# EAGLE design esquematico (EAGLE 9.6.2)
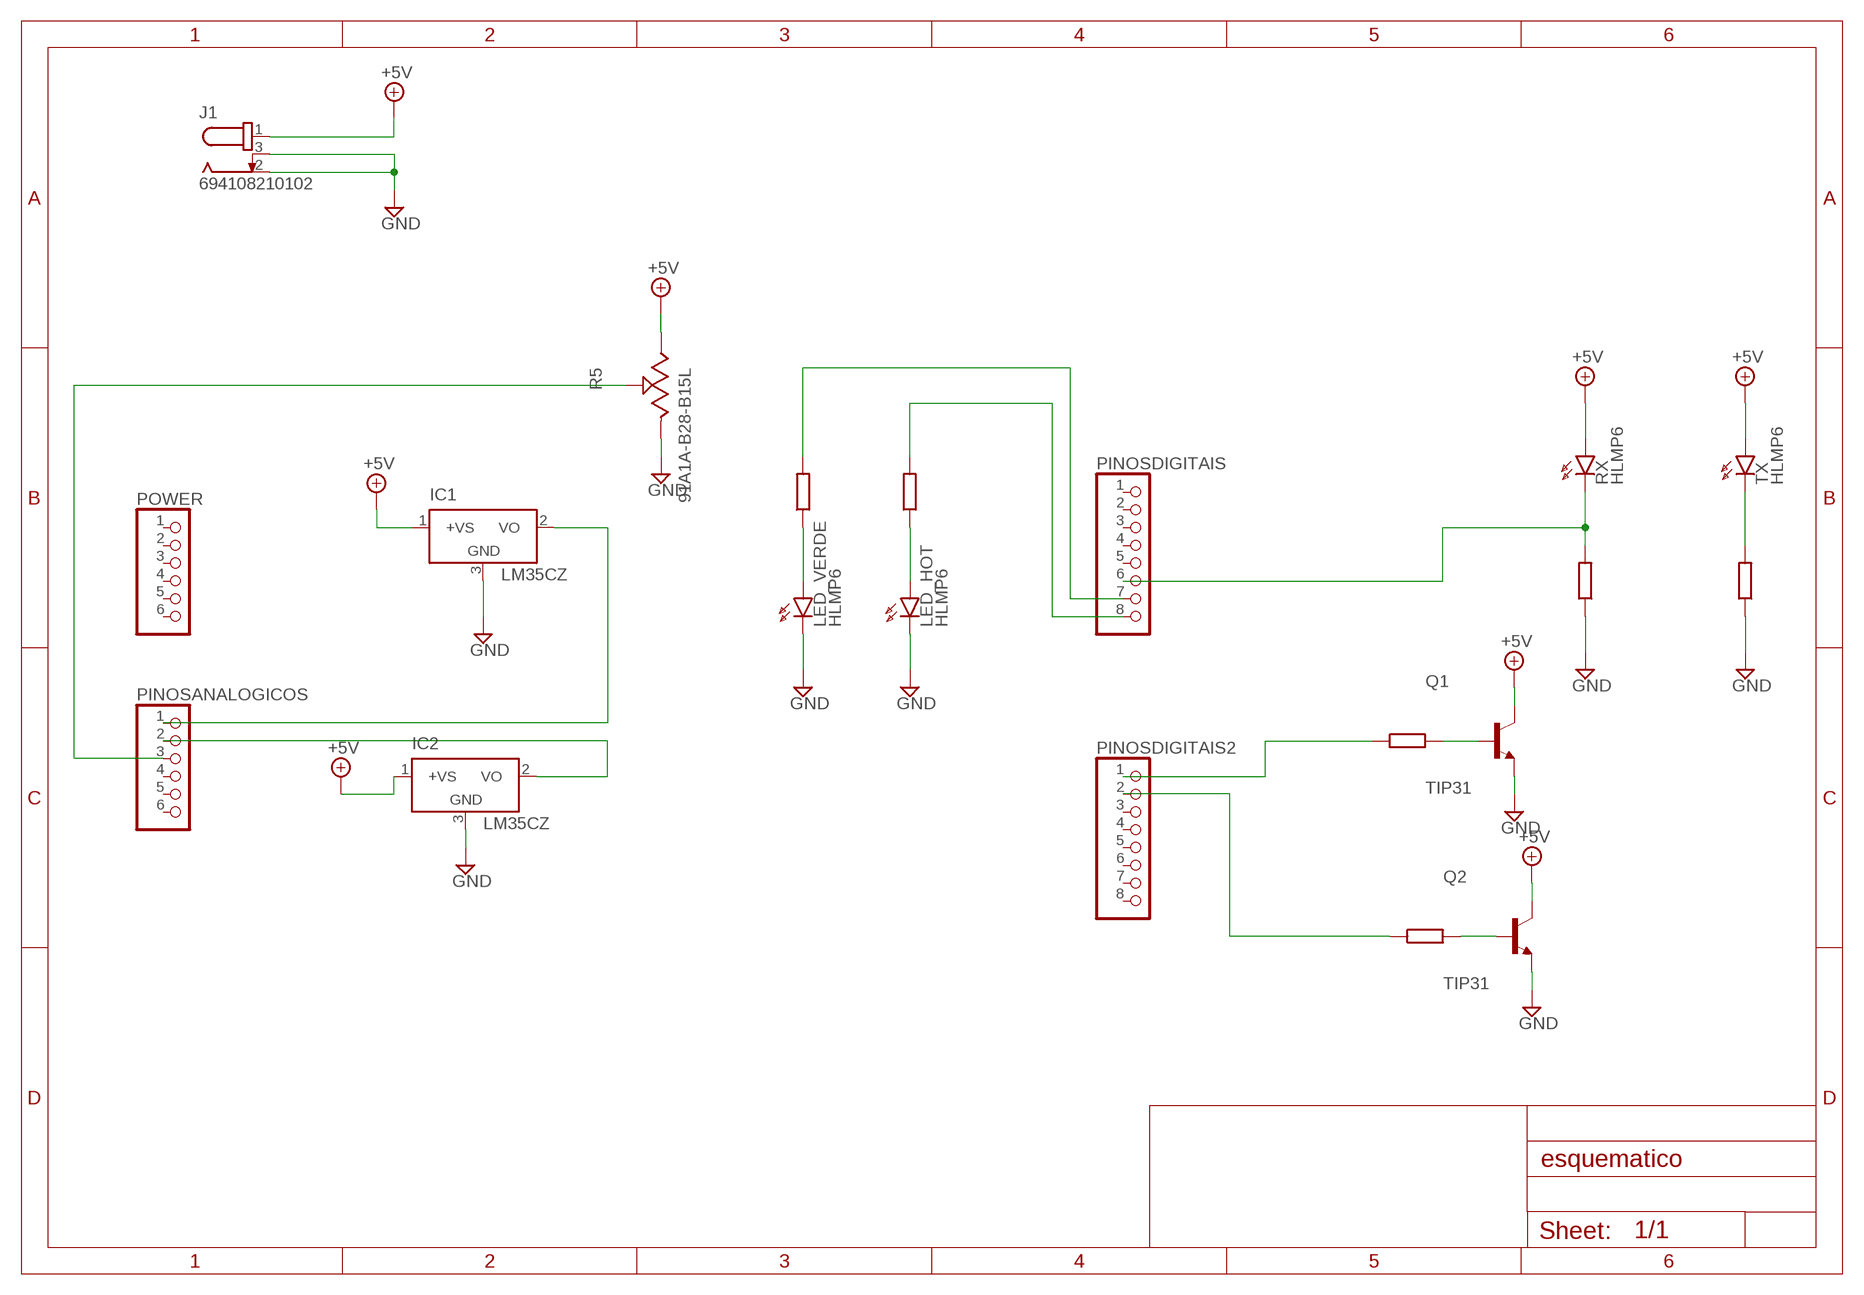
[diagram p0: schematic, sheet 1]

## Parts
IC1  LM35CZ  [TO92]
IC2  LM35CZ  [TO92]
J1  694108210102  [694108210102]
LED_HOT  HLMP6  [HLMP6]
LED_VERDE  HLMP6  [HLMP6]
PINOSANALOGICOS  PINHD-1X6  [1X06]
PINOSDIGITAIS  PINHD-1X8  [1X08]
PINOSDIGITAIS2  PINHD-1X8  [1X08]
POWER  PINHD-1X6  [1X06]
Q1  TIP31  [TO254P1060X482X2222-3]
Q2  TIP31  [TO254P1060X482X2222-3]
R5  91A1A-B28-B15L  [91A1A-B28-B15L-ND]
RX  HLMP6  [HLMP6]
TX  HLMP6  [HLMP6]

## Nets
+5V: IC1.1(+VS) IC2.1(+VS) J1.1 Q1.2(C) Q2.2(C) R5.3 RX.A TX.A
GND: IC1.3(GND) IC2.3(GND) J1.2 J1.3 LED_HOT.K LED_VERDE.K Q1.3(E) Q2.3(E) R5.1
N$1: IC2.2(VO) PINOSANALOGICOS.2
N$2: Q1.1(B)
N$3: LED_HOT.A
N$4: LED_VERDE.A
N$5: IC1.2(VO) PINOSANALOGICOS.1
N$6: Q2.1(B)
N$7: PINOSDIGITAIS2.1
N$8: PINOSDIGITAIS2.2
N$9: PINOSDIGITAIS.6 RX.K
N$10: TX.K
N$11: PINOSDIGITAIS.8
N$12: PINOSDIGITAIS.7
N$13: PINOSANALOGICOS.3 R5.2
Unconnected: PINOSANALOGICOS.4 PINOSANALOGICOS.5 PINOSANALOGICOS.6 PINOSDIGITAIS2.3 PINOSDIGITAIS2.4 PINOSDIGITAIS2.5 PINOSDIGITAIS2.6 PINOSDIGITAIS2.7 PINOSDIGITAIS2.8 PINOSDIGITAIS.1 PINOSDIGITAIS.2 PINOSDIGITAIS.3 PINOSDIGITAIS.4 PINOSDIGITAIS.5 POWER.1 POWER.2 POWER.3 POWER.4 POWER.5 POWER.6

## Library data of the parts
IC1 IC2 = lm35:LM35: Single-Supply Centigrade Temperature Sensor Vout = (10mV/°C x Temp °C) +5mmmV Source: http://www.national.com/ds/LM/LM35.pdf
J1 = DC Power Jacks:694108210102: DC POWER JACK - VERTICAL- THT - Ø 2.0 & 2.5 -WR-DC Manufacturer's datasheet; CREATED_BY: PCBLayout.com; MANUFACTURER: WURTH ELEKTRONIK; MPN: 694108210102
LED_HOT LED_VERDE RX TX = display-hp:HLMP6: LED; MF: AGILENT TECHNOLOGIES; MPN: HLMP-6500; OC_FARNELL: 1652490; OC_NEWARK: 40K0088
PINOSANALOGICOS POWER = pinhead:PINHD-1X6: PIN HEADER
PINOSDIGITAIS PINOSDIGITAIS2 = pinhead:PINHD-1X8: PIN HEADER
Q1 Q2 = TIP31:TIP31: Bipolar (BJT) Transistor NPN 40V 3A 3MHz 2W Through Hole TO-220AB Check prices; AVAILABILITY: In Stock; DESCRIPTION: Bipolar (BJT) Transistor NPN 60V 3A 3MHz 2W Through Hole TO-220AB; MF: ON Semiconductor; MP: TIP31; PACKAGE: TO-220-3 ON Semiconductor; PRICE: None
R5 = Potentiometer_Trimmers:91A1A-B28-B15L: POT 10K OHM 1W PLASTIC LINEAR Manufacturer's datasheet; CREATED_BY: PCBLayout.com; DIGIKEY_PARTNO: 91A1A-B28-B15L-ND; MANUFACTURER: Bourns Inc.; MPN: 91A1A-B28-B15L

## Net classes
0 default: width 0.305 mm, drill 0.305 mm, clearance 0.254 mm

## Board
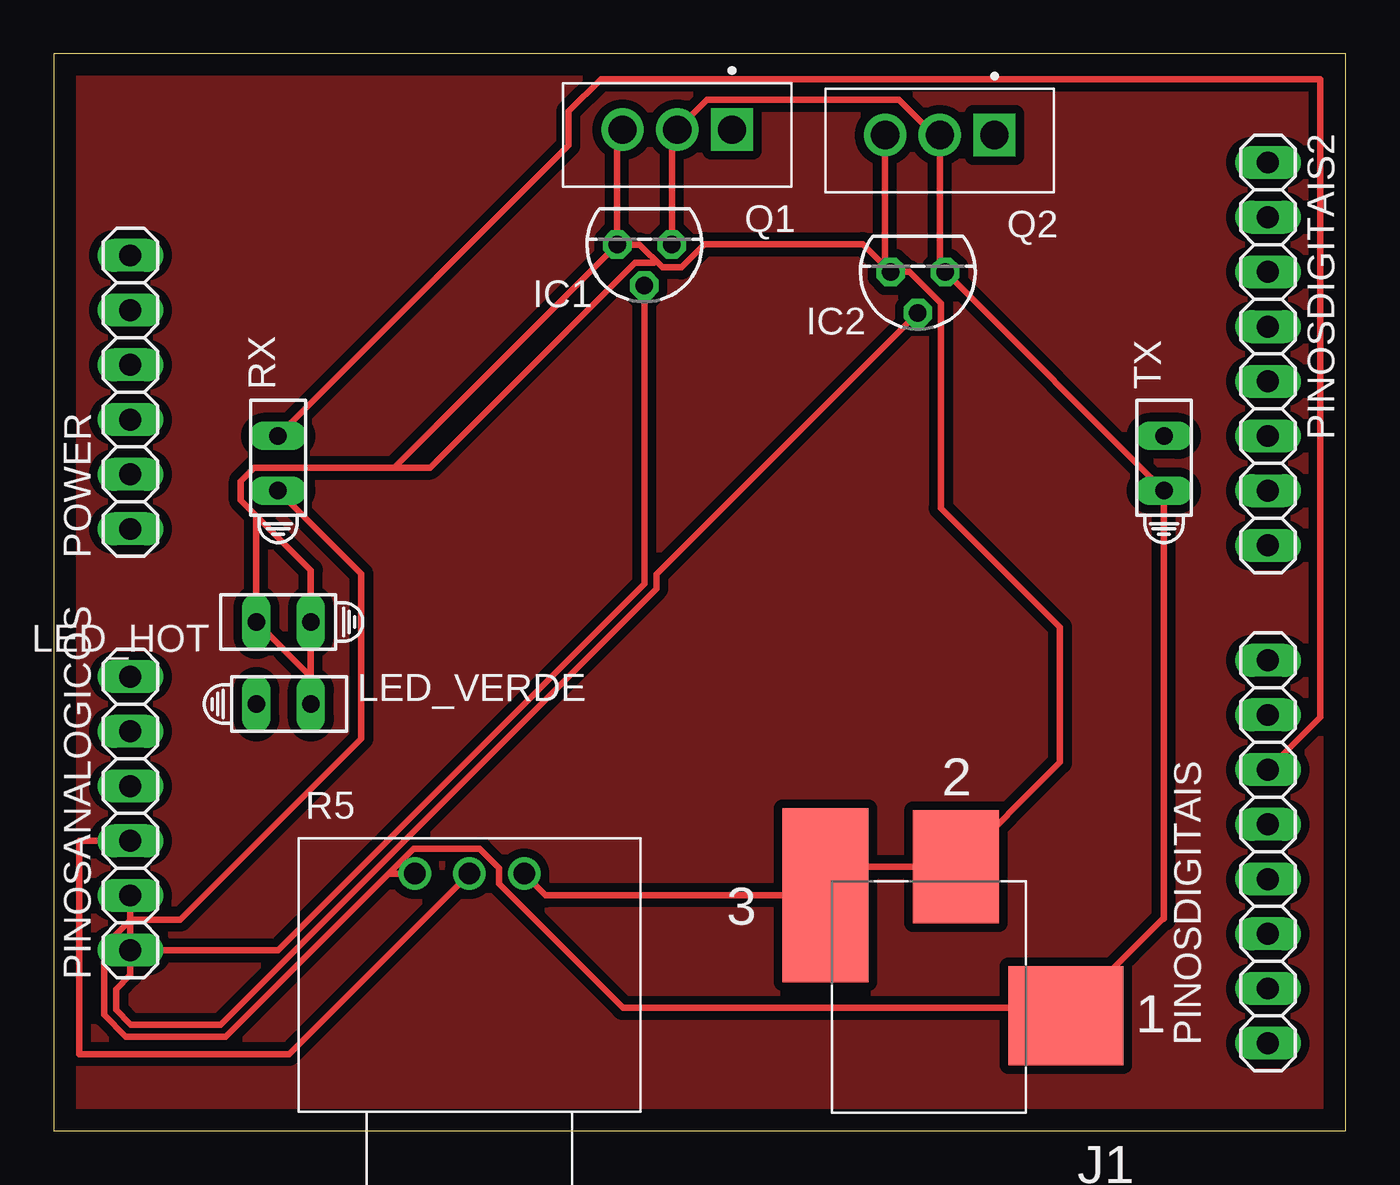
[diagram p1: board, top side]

Size 60 x 50 mm. Coordinates in mm from the lower left corner, seen from the top.
Outline: 0,0 60,0 60,50 0,50 0,0
Copper layers (1*16): Top 0.035mm / dielectric 1.5mm / Bottom 0.035mm
Design rules "default": minimum track width 6mil, minimum drill 0.35mm, track to track 6mil, track to pad 6mil, pad to pad 6mil, via to via 6mil, smd to smd 6mil, copper to edge 40mil, drill to drill 6mil, minimum pad ring 10mil, minimum via ring 8mil, stop-mask expansion 4mil, vias tented up to drill 0mil, thermal gap 10mil

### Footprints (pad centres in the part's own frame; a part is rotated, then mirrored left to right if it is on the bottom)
TO92 = drill 0.813 octagon: 1 -1.27,0; 2 0,1.905; 3 1.27,0
694108210102 = smd 5.33 x 4.6: 1 -6.365,0 | smd 4 x 5.25: 2 -1.25,-6.925 | smd 4 x 8.1: 3 4.8,-5.6
HLMP6 = drill 0.813 long: A -1.27,0; K 1.27,0
1X06 = drill 1.016 long: 1 -6.35,0; 2 -3.81,0; 3 -1.27,0; 4 1.27,0; 5 3.81,0; 6 6.35,0
1X08 = drill 1.016 long: 1 -8.89,0; 2 -6.35,0; 3 -3.81,0; 4 -1.27,0; 5 1.27,0; 6 3.81,0; 7 6.35,0; 8 8.89,0
TO254P1060X482X2222-3 = drill 1.31 square: 1 -2.54,0 | drill 1.31: 2 0,0; 3 2.54,0
91A1A-B28-B15L-ND = drill 1: 1 2.54,0; 2 0,0; 3 -2.54,0

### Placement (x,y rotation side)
IC1  27.43,41.15 180 top
IC2  40.13,39.88 180 top
J1  40.64,5.33 180 top
LED_HOT  10.67,23.62 180 top
LED_VERDE  10.67,19.81 0 top
PINOSANALOGICOS  3.56,14.73 90 top
PINOSDIGITAIS  56.39,12.95 90 top
PINOSDIGITAIS2  56.39,36.07 270 top
POWER  3.56,34.29 90 top
Q1  28.96,46.48 180 top
Q2  41.15,46.23 180 top
R5  19.3,11.94 0 top
RX  10.41,30.99 90 top
TX  51.56,30.99 90 top

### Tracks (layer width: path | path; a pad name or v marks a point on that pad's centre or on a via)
+5V
  Top 0.305: 15.55,11.94 7.98,4.37 3.35,4.37 2.34,5.38 2.34,8.56 3.58,9.8 5.87,9.8 14.28,18.21 14.28,25.86 RX.A | 15.55,11.94 R5.3 | J1.1 47.38,5.71 | 28.98,41.43 IC1.1 28.7,46.23 Q1.2 | 15.55,11.94 16.71,13.1 19.79,13.1 20.68,12.2 20.68,11.46 26.43,5.71 47.38,5.71 | 47.38,5.71 51.53,9.86 51.56,9.84 TX.A IC2.1 41.15,40.13 41.15,45.97 | 41.15,45.97 Q2.2 | Q1.2 | Q1.2 30.34,47.87 39.25,47.87 41.15,45.97
GND
  Top 0.305: R5.1 22.85,10.93 J1.3 37.16,12.26 J1.2 46.74,17.11 46.74,23.37 41.2,28.91 41.2,38.41 39.74,39.88 IC2.3 | 27.87,40.31 26.99,40.31 17.46,30.79 15.8,30.79 | 9.4,28.57 11.94,26.02 LED_VERDE.K 11.94,21.08 LED_HOT.K 9.4,28.57 | 9.4,28.57 8.69,29.28 8.69,30.16 9.31,30.79 15.8,30.79 | 15.8,30.79 IC1.3 | IC1.3 27.19,41.15 28.26,40.08 29.14,40.08 30.23,41.16 37.58,41.16 IC2.3 | IC1.3 26.16,46.23 Q1.3 | IC2.3 38.61,40.13 Q2.3
N$1
  Top 0.305: IC2.2 27.99,25.83 27.99,25.17 7.75,4.93 3.58,4.93 2.9,5.61 2.9,6.58 3.56,7.24 PINOSANALOGICOS.2
N$5
  Top 0.305: PINOSANALOGICOS.1 10.41,8.38 27.43,25.4 IC1.2
N$9
  Top 0.305: RX.K 23.9,45.74 23.9,47.33 25.41,48.83 58.83,48.83 58.83,19.21 PINOSDIGITAIS.6
N$13
  Top 0.305: R5.2 10.92,3.56 1.17,3.56 1.17,13.46 PINOSANALOGICOS.3
PLANO_DE_TERRA
  pour Top (isolate 0.406): 0.25,49.78 59.69,49.78 59.69,45.47 59.69,0.25 0.25,0.25 0.25,1.02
